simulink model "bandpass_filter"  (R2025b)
settings: Solver=VariableStepDiscrete  StartTime=0.0  StopTime=inf  RelTol=1e-3  EnableMultiTasking=on
undefined symbols (not defined in the file or in its folder): gateway_in_config, gateway_out_config, hex2dec, netlist, Register_config, sysgen
libraries: hdlBasic x4, dspsrcs4 x1, dspobslib x1, vmcUtilities x1

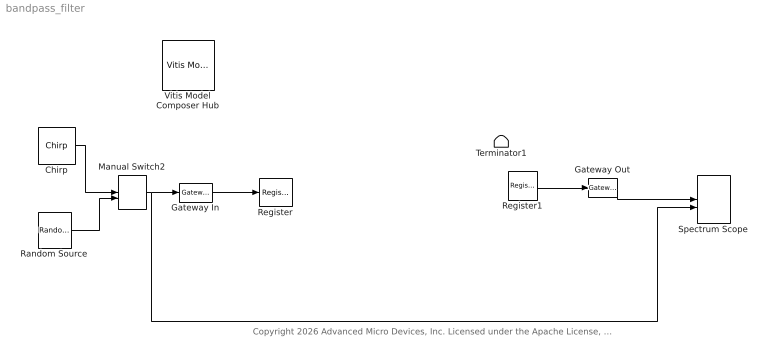
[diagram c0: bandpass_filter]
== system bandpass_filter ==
  note: Copyright 2026 Advanced Micro Devices, Inc. Licensed under the Apache License, Version 2.0 (the "License"); you may not use this file except in compliance with the License. You may obtain a copy of the License at http://www.apache.org/licenses/LICENSE-2.0 Unless required by applicable law or agreed to in writing, software distributed under the License is distributed on an "AS IS" BASIS, WITHOUT WARRANTIES OR CONDITIONS OF ANY KIND, either express or implied. See the License for the specific language governing permissions and limitations under the License.
  Chirp : dspsrcs4/Chirp  sweep=Swept cosine  mode=Bidirectional  f0=300000  f1=800000  t1=0.01  Tsweep=0.01  phase=0  Ts=1/3000000  spf=1  datatype=double  OutputFrames=on
  Gateway In : hdlBasic/Gateway In  gui_display_data_type=Fixed-point  arith_type=Signed (2's comp)  n_bits=16  bin_pt=12  preci_type=Single  exp_width=8  frac_width=24  rows=1  columns=1  quantization="Round  (unbiased: +/- Inf)"  overflow=Saturate  period=1  UseAsADC=off  ADCChannel='1'  interface=None  automatic_assignment=on  address_offset=hex2dec('00')  intf_name=''  intf_description=''  default_value=0  timing_constraint=None  locs_specified=off  LOCs={}  io_standard={}  inherit_from_input=off  hdl_port=on  XmcBlockStatus=1  maskContainerNames=group4  block_type=gatewayin  block_config=sysgen:gateway_in_config  block_width_w=590  block_height_w=620  block_width=640  block_height=850
  Gateway Out : hdlBasic/Gateway Out  inherit_from_input=off  bool_to_boolean=off  hdl_port=on  rows=1  columns=1  UseAsDAC=off  DACChannel='1'  interface=None  automatic_assignment=on  address_offset=hex2dec('00')  intf_name=''  intf_description=''  timing_constraint=None  locs_specified=off  LOCs={}  io_standard={}  XmcBlockStatus=1  maskContainerNames=group4  block_type=gatewayout  block_config=sysgen:gateway_out_config  block_width_w=590  block_height_w=620  block_width=620  block_height=750
  Manual Switch2 : ManualSwitch
  Random Source : dspobslib/Random Source  SrcType=Uniform  NormMethod=Ziggurat  CltLength=12  MinVal=-1  MaxVal=1  MeanVal=0  VarVal=1  RepMode=Not repeatable  rawSeed=1  IsInherit=off  SampMode=Discrete  SampTime=1/3000000  SampFrame=1  DataType=Double  OutComplex=Real  OutputFrames=on
  Register : hdlBasic/Register  init=0  rst=off  en=off  XmcBlockStatus=1  maskContainerNames=tabcontainer1  block_type=register  block_config=sysgen:Register_config
  Register1 : hdlBasic/Register  init=0  rst=off  en=on  XmcBlockStatus=1  maskContainerNames=tabcontainer1  block_type=register  block_config=sysgen:Register_config
  Spectrum Scope : SpectrumAnalyzer  NumInputPorts=2  WindowPosition=[75.000000,1.000000,1846.000000,902.000000,]  ScopeFrameLocation=window  Method=Welch  SampleRate=3000000  PlotAsTwoSidedSpectrum=off  AxesScaling=Manual  FrequencyResolutionMethod=Window length  WindowLength=512  FFTLengthSource=Property  FFTLength=512  Span=1500000  CenterFrequency=750000  StartFrequency=0  StopFrequency=1500000  OverlapPercent=50  AveragingMethod=Running  SpectralAverages=2  YLabel=Magnitude-squared  YLimits=[-146,44]  ShowGrid=off  AllowFFTLengthLessThanSamplesPerUpdate=on  SegLen=512
  Terminator1 : Terminator
  Vitis Model Composer Hub : vmcUtilities/Vitis Model Composer Hub  Tag=genX  CodeGeneration=off  CompilationType=HDLCompilation  ExportTypeV2=IP Catalog  StartColumn=1  NumberOfColumns=1  TargetDirectory=./netlist  exportDesign=off  analyzeDesign=off  validateDesignOnHw=off  ExportType=AI Engines  IpVendor=xilinx.com  IpLibrary=hls  IpVersion=1.0  IpHWLanguage=Verilog  AieCompilerOptions={}  AieSimulatorOptions={}  CreateTestbench=off  TestbenchStackSize=10  RunRtlSim=off  RunCSim=off  RunAieSim=off  AieSimTimeout=50000  RunAieSimProfiling=off  LaunchVitisAnalyzer=off  PlotOutput=off  RunX86Sim=off  X86SimTimeout=10  GenHwImage=off  GenLibadfXo=off  GenHwValidationCode=off  PlatformType=Not Specified  HwSystemType=Baremetal  HwValidationTarget=hw  SamplePeriod=-1  ClockFrequency=200  DataPathParallelism=1  xilinxfamily=Kintex7  part=xc7k325t  speed=-3  package=fbg676  directory=./netlist  testbench=off  incr_netlist=off  synthesis_tool=Vivado  clock_wrapper=Clock Enables  dbl_ovrd=According to Block Masks  dcm_input_clock_period=10  sysclk_period=10  simulink_period=1  eval_field=0  LogFileName=''  NThreads=4
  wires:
  Gateway In/1 -> Register/1
  Gateway Out/1 -> Spectrum Scope/1
  Manual Switch2/1 -> Spectrum Scope/2, Gateway In/1
  Chirp/1 -> Manual Switch2/1
  Random Source/1 -> Manual Switch2/2
  Register/1 -> ?
  Register1/1 -> Gateway Out/1
  ? -> Terminator1/1
  ? -> Register1/1
  ? -> Register1/2
